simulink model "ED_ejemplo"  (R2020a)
settings: Solver=VariableStepAuto  StartTime=0.0  StopTime=50  RelTol=1e-3
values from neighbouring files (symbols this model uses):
  b = 0.1    [Comando_linmod.m]
  k = 0.8    [Comando_linmod.m]
  kf = 0.45    [Comando_linmod.m]
  kv = 0.45    [Comando_linmod.m]
  L = 0.1    [Comando_linmod.m]
  m = 0.15    [Comando_linmod.m]
  M = 5    [Comando_linmod.m]
  R = 0.25    [Comando_linmod.m]

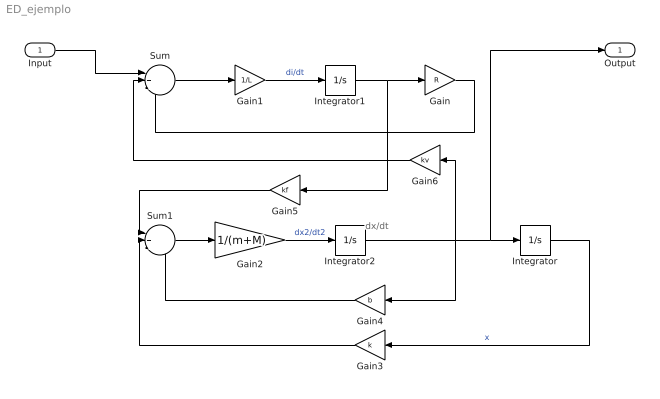
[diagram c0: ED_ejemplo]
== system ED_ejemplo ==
  note: dx/dt
  Input : Inport
  Gain : Gain  Gain=R
  Gain1 : Gain  Gain=1/L
  Gain2 : Gain  Gain=1/(m+M)
  Gain3 : Gain  Gain=k
  Gain4 : Gain  Gain=b
  Gain5 : Gain  Gain=kf
  Gain6 : Gain  Gain=kv
  Integrator : Integrator
  Integrator1 : Integrator
  Integrator2 : Integrator
  Sum : Sum  Inputs=|+--
  Sum1 : Sum  Inputs=|+--
  Output : Outport
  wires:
  Integrator1/1 -> Gain5/1, Gain/1  "i"
  Gain/1 -> Sum/3
  Sum/1 -> Gain1/1
  Gain1/1 -> Integrator1/1  "di/dt"
  Sum1/1 -> Gain2/1
  Gain2/1 -> Integrator2/1  "dx2/dt2"
  Integrator2/1 -> Gain4/1, Gain6/1, Output/1, Integrator/1
  Gain4/1 -> Sum1/3
  Integrator/1 -> Gain3/1  "x"
  Gain3/1 -> Sum1/2
  Gain6/1 -> Sum/2
  Gain5/1 -> Sum1/1
  Input/1 -> Sum/1
